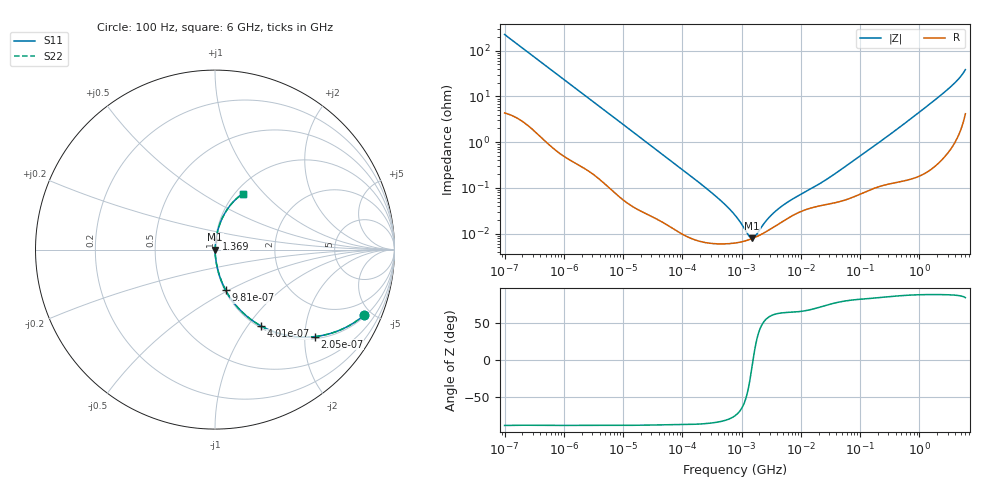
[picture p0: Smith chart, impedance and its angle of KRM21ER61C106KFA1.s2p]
!Murata Part Number: KRM21ER61C106KFA1
!These Parameters are Measured in Series Mode Connection
!Data Generated on Jan 08, 2026
!  o--ll--o
!Port1  Port2
!  o------o
!Operation Temp=25[degC], DC Bias Voltage=0[V]
!Freq. Start=100[Hz] Stop=6[GHz] 401[Steps]
# Hz S RI R 50
!Freq.(Hz) S11(Real) S11(Imag) S21(Real) S21(Imag) S12(Real) S12(Imag) S22(Real) S22(Imag)
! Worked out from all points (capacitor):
!   401 points, 100 Hz to 6 GHz, reference 50 ohm
!   read as one part in series: C = 6.97 uF near 109 Hz
!   lowest |Z| = 7.82 mohm at 1.516 MHz (marker M1)
!   series resonance near 1.565 MHz, so ESL is about 1.5 nH
!   S11 on the Smith chart (normalised r, x): 100 Hz: 1.09, -4.54; 205 Hz: 1.06, -2.25; 401 Hz: 1.03, -1.16; 981 Hz: 1.01, -0.48; 1.369 GHz: 1.00, +0.12; 6 GHz: 1.08, +0.77
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100  0.8328 -0.3636  0.1672 0.3636  0.1672 0.3636  0.8328 -0.3636
137  0.7312 -0.4322  0.2688 0.4322  0.2688 0.4322  0.7312 -0.4322
205  0.5572 -0.4845  0.4428 0.4845  0.4428 0.4845  0.5572 -0.4845
401  0.2579 -0.4263  0.7421 0.4263  0.7421 0.4263  0.2579 -0.4263
627  0.1278 -0.3237  0.8722 0.3237  0.8722 0.3237  0.1278 -0.3237
981  0.0586 -0.2248  0.9414 0.2248  0.9414 0.2248  0.0586 -0.2248
2008  0.0166 -0.116  0.9834 0.116  0.9834 0.116  0.0166 -0.116
6433  0.00231 -0.0376  0.9977 0.0376  0.9977 0.0376  0.00231 -0.0376
40335  0.000233 -0.00615  0.9998 0.00615  0.9998 0.00615  0.000233 -0.00615
316350  6.11e-05 -0.000769  0.9999 0.000769  0.9999 0.000769  6.11e-05 -0.000769
774597  6.19e-05 -0.000245  0.9999 0.000245  0.9999 0.000245  6.19e-05 -0.000245
1212075  7.02e-05 -8.15e-05  0.9999 8.15e-05  0.9999 8.15e-05  7.02e-05 -8.15e-05
1516199  7.76e-05 -9.8e-06  0.9999 9.8e-06  0.9999 9.8e-06  7.76e-05 -9.8e-06
1896632  8.82e-05 5.9e-05  0.9999 -5.9e-05  0.9999 -5.9e-05  8.82e-05 5.9e-05
2967816  0.000121 0.000196  0.9999 -0.000196  0.9999 -0.000196  0.000121 0.000196
4643984  0.000175 0.000344  0.9998 -0.000344  0.9998 -0.000344  0.000175 0.000344
1.555665e7  0.000368 0.000915  0.9996 -0.000915  0.9996 -0.000915  0.000368 0.000915
3.80911e7  0.000476 0.00199  0.9995 -0.00199  0.9995 -0.00199  0.000476 0.00199
3.124326e8  0.00142 0.0143  0.9986 -0.0143  0.9986 -0.0143  0.00142 0.0143
1.369159e9  0.00603 0.0615  0.994 -0.0615  0.994 -0.0615  0.00603 0.0615
3.666503e9  0.0384 0.1706  0.9616 -0.1706  0.9616 -0.1706  0.0384 0.1706
6e9  0.155 0.3116  0.845 -0.3116  0.845 -0.3116  0.155 0.3116
